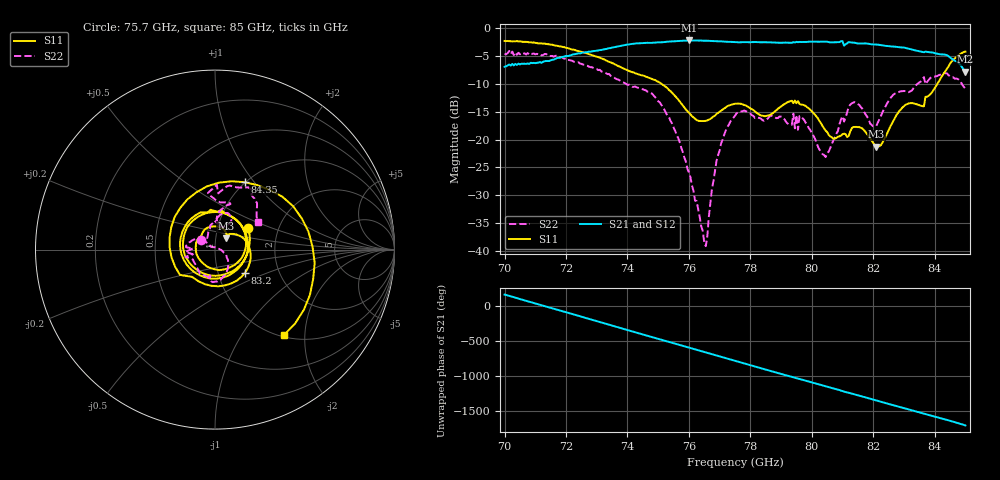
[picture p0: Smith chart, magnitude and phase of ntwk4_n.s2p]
! RsaToolbox (C) 2015 Rohde & Schwarz America
! Number of points: 301
! Number of ports: 2
! Balanced ports?: No
# Hz S RI R 50
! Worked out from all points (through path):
!   301 points, 70 GHz to 85 GHz, reference 50 ohm
!   highest |S21| = -2.27 dB at 76 GHz (marker M1); lowest = -7.8 dB at 85 GHz (marker M2)
!   lowest |S11| = -21.3 dB at 82.1 GHz (marker M3), VSWR 1.19, Z = 55.8 + j7.04 ohm
!   |S11| at or under -10 dB: 75.09 GHz to 84.09 GHz (8.997 GHz wide, 11.3 % of centre)
!   |S22| runs from -39.1 to -4.1 dB; largest |S21 - S12| = 0
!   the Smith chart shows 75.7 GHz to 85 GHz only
!   S11 on the Smith chart (normalised r, x): 75.7 GHz: 1.40, +0.35; 83.2 GHz: 1.35, -0.36; 84.35 GHz: 0.99, +0.90; 85 GHz: 1.03, -1.57
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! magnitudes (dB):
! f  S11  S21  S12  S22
! 70 GHz  -2.4  -7.0  -7.0  -4.6
! 72.5 GHz  -4.3  -4.5  -4.5  -6.5
! 75 GHz  -9.7  -2.6  -2.6  -13.2
! 75.7 GHz  -13.2  -2.4  -2.4  -20.5
! 76 GHz  -15.2  -2.3  -2.3  -25.9
! 76.55 GHz  -16.6  -2.3  -2.3  -39.1
! 76.9 GHz  -15.4  -2.4  -2.4  -23.8
! 77.5 GHz  -13.6  -2.6  -2.6  -15.8
! 78.5 GHz  -15.8  -2.6  -2.6  -16.6
! 79.35 GHz  -13.1  -2.7  -2.7  -17.4
! 79.4 GHz  -13.5  -2.6  -2.6  -15.4
! 79.45 GHz  -13.0  -2.6  -2.6  -18.0
! 79.65 GHz  -13.8  -2.6  -2.6  -15.8
! 80 GHz  -15.0  -2.5  -2.5  -18.8
! 80.45 GHz  -18.4  -2.5  -2.5  -23.2
! 81.4 GHz  -17.8  -2.7  -2.7  -13.3
! 82.1 GHz  -21.3  -3.0  -3.0  -17.6
! 82.5 GHz  -18.4  -3.3  -3.3  -13.1
! 83.2 GHz  -13.5  -3.8  -3.8  -11.4
! 83.65 GHz  -14.1  -4.4  -4.4  -8.8
! 84.35 GHz  -7.7  -4.8  -4.8  -8.1
! 85 GHz  -4.3  -7.8  -7.8  -10.9
